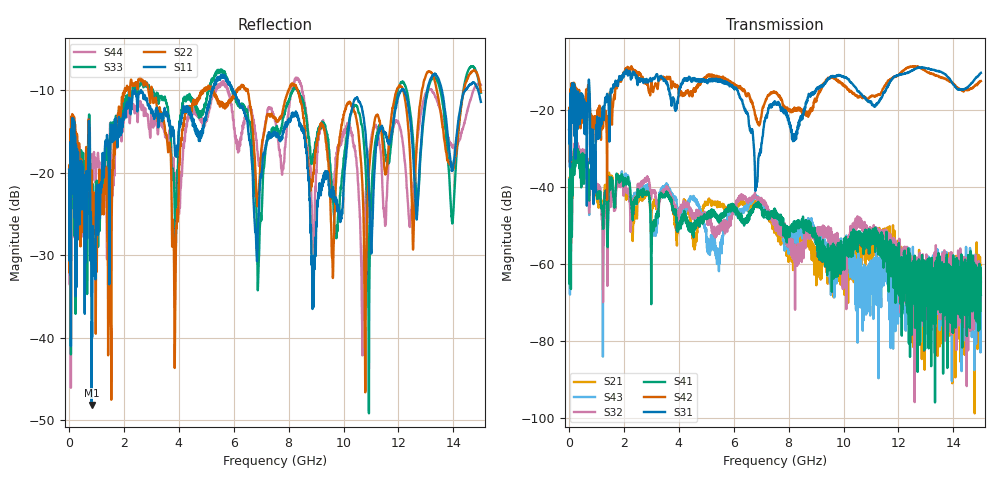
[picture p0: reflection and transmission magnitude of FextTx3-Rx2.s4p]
! FILE: N:\QM 2007\Prüfprotokolle\Highspeed\Konfektionierte Ltg\L45593-D106\D30\8216\0002\Fext\FextTx3-Rx2.s4p
# MHz S RI R 50.00
! FREQ  S11  S12  S13  S14
!  S21  S22  S23  S24
!  S31  S32  S33  S34
!  S41  S42  S43  S44
!  REAL  IMAG  REAL  IMAG  REAL  IMAG  REAL  IMAG
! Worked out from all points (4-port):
!   2999 points, 10 MHz to 15 GHz, reference 50 ohm
!   strongest paths, dB at 10 MHz, 3.755 GHz, 7.505 GHz, 11.26 GHz, 15 GHz:
!     S31: -24.9, -17.2, -18.1, -18.1, -10.3
!     S42: -24.9, -13.0, -15.3, -16.0, -12.4
!     S41: -41.2, -45.0, -45.6, -51.8, -67.9
!     S32: -47.5, -43.4, -49.3, -51.6, -64.7
!     S43: -42.2, -42.2, -47.9, -58.3, -64.1
!     S21: -43.3, -44.5, -50.1, -56.4, -63.4
!   lowest |S11| = -48.2 dB at 830 MHz (marker M1), VSWR 1.01, Z = 49.8 + j0.318 ohm
!   |S11| at or under -10 dB: start of sweep to 2.397 GHz; 2.626 GHz to 5.221 GHz (2.594 GHz wide, 66.1 % of centre); 5.966 GHz to 12.11 GHz (6.141 GHz wide, 68 % of centre)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
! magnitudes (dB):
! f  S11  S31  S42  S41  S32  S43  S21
! 10 MHz  -19.6  -24.9  -24.9  -41.2  -47.5  -42.2  -43.3
! 830 MHz  -48.2  -29.1  -21.5  -34.3  -33.6  -33.3  -34.7
! 2.145 GHz  -11.9  -10.7  -9.0  -37.9  -40.6  -36.9  -41.9
! 8.305 GHz  -12.8  -26.0  -20.1  -49.4  -56.9  -51.2  -57.4
! 8.895 GHz  -32.1  -15.8  -19.4  -51.1  -52.9  -50.7  -55.1
! 10.69 GHz  -12.6  -16.3  -16.8  -52.7  -49.0  -62.6  -55.9
! 15 GHz  -11.4  -10.3  -12.4  -67.9  -64.7  -64.1  -63.4
